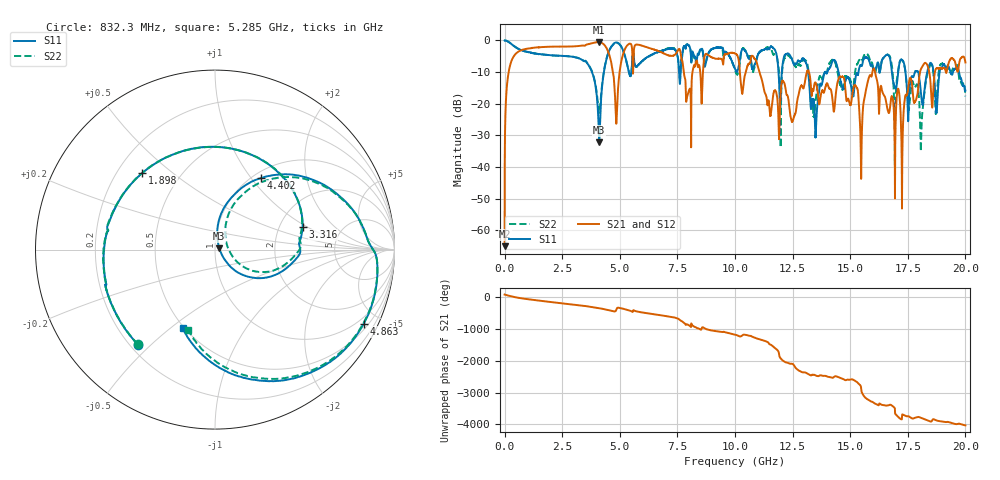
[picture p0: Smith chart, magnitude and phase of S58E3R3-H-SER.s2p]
!{S58E3R3}
!Johanson Technology Inc.
!www.johansontechnology.com
!Test Board Conditions:
!Substrate Type  RO4350B
!Substrate Thickness  60 mil
!Substrate Dk  3.66
!TL Type: GCPW
!TL Trace Width  115 mil
!TL Gap  52 mil
!Electrode orientation  Horizontal
!DUT TOPOLOGY	SERIES
!Mounting Pad LxW  55x428 mil
! Created Tue Apr 13 22:37:11 2021
# hz S ma R 50
! 2 Port Network Data from SP1.SP block
! freq  magS11  angS11  magS21  angS21  magS12  angS12  magS22  angS22
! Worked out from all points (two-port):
!   20001 points, 300 kHz to 20 GHz, reference 50 ohm
!   highest |S21| = -0.54 dB at 4.081 GHz (marker M1); lowest = -65.0 dB at 300 kHz (marker M2)
!   |S21| within 3 dB of the highest: 597.2 MHz to 4.497 GHz (3.9 GHz wide, 153 % of centre); 5.606 GHz to 6.743 GHz (1.136 GHz wide, 18.4 % of centre)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
!   lowest |S11| = -32.1 dB at 4.108 GHz (marker M3), VSWR 1.05, Z = 52.4 + j0.821 ohm
!   |S11| at or under -10 dB: 3.797 GHz to 4.31 GHz (512.8 MHz wide, 12.7 % of centre); 13.17 GHz to 13.9 GHz (720.9 MHz wide, 5.33 % of centre); 14.49 GHz to 15.36 GHz (867.9 MHz wide, 5.81 % of centre)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
!   |S22| runs from -39.4 to 0.0 dB; largest |S21 - S12| = 0.0082
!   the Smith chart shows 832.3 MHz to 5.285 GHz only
!   S11 on the Smith chart (normalised r, x): 832.3 MHz: 0.23, -0.46; 1.898 GHz: 0.30, +0.40; 3.316 GHz: 2.68, +0.91; 4.402 GHz: 1.09, +1.12; 4.863 GHz: 0.71, -4.13; 5.285 GHz: 0.49, -0.55
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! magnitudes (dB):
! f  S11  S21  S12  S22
! 300 kHz  0.0  -65.0  -64.5  0.0
! 175.3 MHz  -0.5  -10.0  -10.0  -0.5
! 832.3 MHz  -3.3  -2.8  -2.8  -3.3
! 1.898 GHz  -4.6  -2.0  -2.0  -4.6
! 3.316 GHz  -5.9  -1.7  -1.7  -5.9
! 3.334 GHz  -6.0  -1.6  -1.6  -6.0
! 4.081 GHz  -27.4  -0.5  -0.6  -22.1
! 4.108 GHz  -32.1  -0.6  -0.6  -22.9
! 4.402 GHz  -6.5  -2.1  -2.1  -6.3
! 4.863 GHz  -0.7  -24.6  -24.6  -0.7
! 5.285 GHz  -6.5  -1.9  -1.9  -6.6
! 6.667 GHz  -3.6  -3.3  -3.3  -3.7
! 8.005 GHz  -1.7  -15.7  -15.6  -1.7
! 10 GHz  -8.9  -4.1  -4.1  -9.2
! 12.49 GHz  -6.4  -25.5  -25.6  -6.0
! 13.33 GHz  -18.8  -17.4  -17.5  -19.4
! 16.67 GHz  -4.7  -22.9  -22.8  -4.6
! 16.95 GHz  -14.9  -40.8  -42.1  -29.0
! 17.27 GHz  -6.2  -34.0  -33.8  -6.4
! 18.09 GHz  -17.7  -8.8  -8.8  -29.6
! 18.48 GHz  -7.1  -12.8  -12.8  -7.7
! 20 GHz  -15.8  -7.0  -6.9  -17.7
